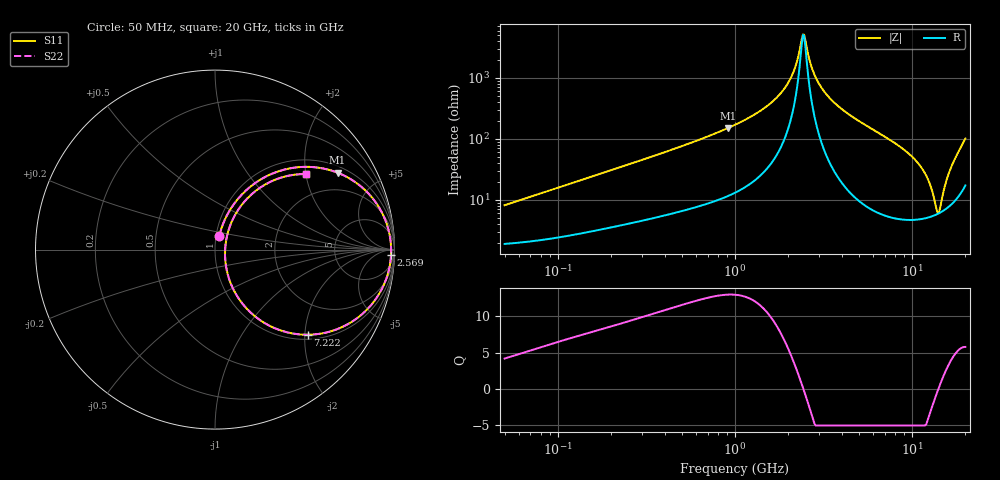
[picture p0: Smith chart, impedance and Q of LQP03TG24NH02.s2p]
!Murata Part Number: LQP03TG24NH02
!These Parameters are Measured in Series Mode Connection
!  o--[Z]--o
!Port1  Port2
!  o-------o
!Freq. Start=50[MHz] Stop=20[GHz], 401[Steps]
# Hz S RI R 50
!Freq.(Hz) S11(Real) S11(Imag) S21(Real) S21(Imag) S12(Real) S12(Imag) S22(Real) S22(Imag)
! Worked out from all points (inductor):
!   401 points, 50 MHz to 20 GHz, reference 50 ohm
!   read as one part in series: L = 25.2 nH near 51.52 MHz
!   highest Q = 13 at 914 MHz (marker M1), where L = 26.3 nH
!   self-resonance near 2.42 GHz
!   S11 on the Smith chart (normalised r, x): 50 MHz: 1.04, +0.16; 2.569 GHz: 28, -47; 7.222 GHz: 1.11, -2.07; 20 GHz: 1.35, +2.01
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5e7  0.0246 0.0764  0.9754 -0.0764  0.9754 -0.0764  0.0246 0.0764
1.364002e8  0.0671 0.1918  0.9329 -0.1918  0.9329 -0.1918  0.0671 0.1918
3.721004e8  0.2602 0.3941  0.7398 -0.3941  0.7398 -0.3941  0.2602 0.3941
9.140482e8  0.6831 0.4283  0.3169 -0.4283  0.3169 -0.4283  0.6831 0.4283
1e9  0.7288 0.4077  0.2712 -0.4077  0.2712 -0.4077  0.7288 0.4077
1.432596e9  0.8838 0.2789  0.1162 -0.2789  0.1162 -0.2789  0.8838 0.2789
1.848039e9  0.9532 0.1535  0.0468 -0.1535  0.0468 -0.1535  0.9532 0.1535
2.146657e9  0.9749 0.0716  0.0251 -0.0716  0.0251 -0.0716  0.9749 0.0716
2.419936e9  0.9813 0.00352  0.0187 -0.00352  0.0187 -0.00352  0.9813 0.00352
2.569357e9  0.9808 -0.031  0.0192 0.031  0.0192 0.031  0.9808 -0.031
2.728004e9  0.9776 -0.0657  0.0224 0.0657  0.0224 0.0657  0.9776 -0.0657
3.121702e9  0.9607 -0.1436  0.0393 0.1436  0.0393 0.1436  0.9607 -0.1436
3.792786e9  0.9109 -0.2528  0.0891 0.2528  0.0891 0.2528  0.9109 -0.2528
7.222371e9  0.5159 -0.4744  0.4841 0.4744  0.4841 0.4744  0.5159 -0.4744
7.442007e9  0.4899 -0.4738  0.5101 0.4738  0.5101 0.4738  0.4899 -0.4738
1.115139e10  0.1436 -0.2889  0.8564 0.2889  0.8564 0.2889  0.1436 -0.2889
1.238412e10  0.0827 -0.1755  0.9173 0.1755  0.9173 0.1755  0.0827 -0.1755
1.396067e10  0.056 -0.0116  0.944 0.0116  0.944 0.0116  0.056 -0.0116
1.438523e10  0.0595 0.034  0.9405 -0.034  0.9405 -0.034  0.0595 0.034
1.550395e10  0.0918 0.1522  0.9082 -0.1522  0.9082 -0.1522  0.0918 0.1522
1.670968e10  0.1639 0.2675  0.8361 -0.2675  0.8361 -0.2675  0.1639 0.2675
2e10  0.5076 0.421  0.4924 -0.421  0.4924 -0.421  0.5076 0.421
